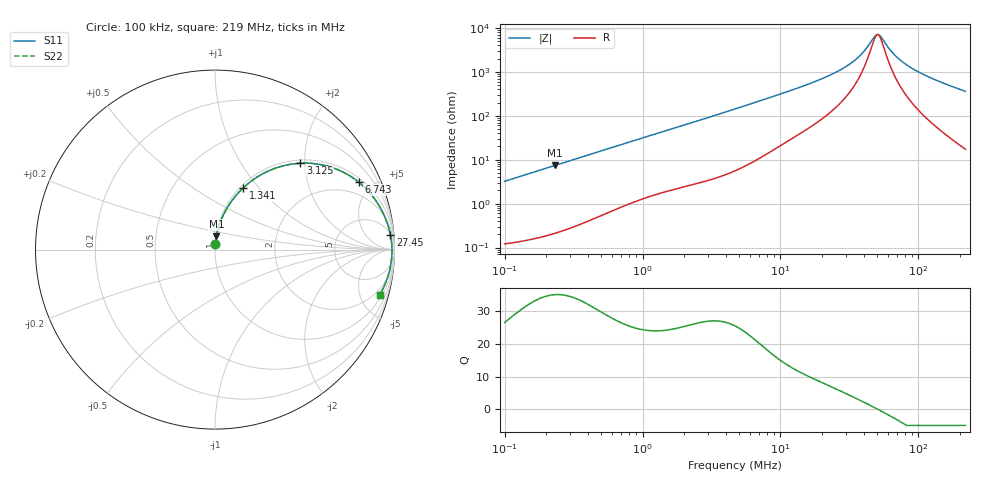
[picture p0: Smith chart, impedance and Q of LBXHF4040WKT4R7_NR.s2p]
! LBXHF4040WKT4R7_NR  S-PARAMETER MODEL  ( General Type )
! Model Generated by TAIYO YUDEN Corporation (http://www.ty-top.com)
! Version 1.0
! TAIYO YUDEN Control No. 210719NI43SB-FBB
! Copyright(c) 2021 TAIYO YUDEN CO.,LTD. All Rights Reserved.
! Product Description (link to TY-COMPAS)
! https://ds.yuden.co.jp/TYCOMPAS/or/detail?pn=LBXHF4040WKT4R7MNR&u=M
! Products Name : Inductors
! Characteristics :
!  Inductance : 4.7 uH , SRF(min) : 36 MHz , DC Resistance(max) : 0.084 Ohm
!  Rated Current : Saturation :2000 mA , Temp Rise : 1500 mA
!  Case Size : 4.0 x 4.0 / 0.157 x 0.157 [mm/inch] , Thickness : 2 / 0.079 [mm/inch]
!  (Conditions: Temperature = 25 degC , DC Bias Current/Voltage = 0A / 0V)
! External Node Assignments :
!  1  o---GGG---o  2
! GND o---------o GND
! Frequency Range : 0.1MHz  -  218.972167MHz  [ 402 STEP ]
# MHz S RI R 50
! Freq[MHz].  S11 Real  S11 Imag  S21 Real  S21 Imag  S12 Real  S12 Imag  S22 Real  S22 Imag
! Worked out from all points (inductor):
!   401 points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, 100 kHz to 219 MHz, reference 50 ohm
!   read as one part in series: L = 5.11 uH near 103.9 kHz
!   highest Q = 35.2 at 233 kHz (marker M1), where L = 5.09 uH
!   self-resonance near 49.82 MHz
!   S11 on the Smith chart (normalised r, x): 100 kHz: 1.00, +0.06; 1.341 MHz: 1.03, +0.83; 3.125 MHz: 1.07, +1.90; 6.743 MHz: 1.20, +4.14; 27.45 MHz: 5, +22; 219 MHz: 1.35, -7.18
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0.1  0.00224 0.0321  0.9978 -0.0321  0.9978 -0.0321  0.00224 0.0321
0.233047  0.00761 0.0739  0.9924 -0.0739  0.9924 -0.0739  0.00761 0.0739
0.362673  0.0165 0.1133  0.9835 -0.1133  0.9835 -0.1133  0.0165 0.1133
0.753099  0.0607 0.2202  0.9393 -0.2202  0.9393 -0.2202  0.0607 0.2202
1.315317  0.1518 0.3386  0.8482 -0.3386  0.8482 -0.3386  0.1518 0.3386
1.340853  0.1564 0.343  0.8436 -0.343  0.8436 -0.343  0.1564 0.343
2.007944  0.2811 0.4302  0.7189 -0.4302  0.7189 -0.4302  0.2811 0.4302
3.124813  0.475 0.4812  0.525 -0.4812  0.525 -0.4812  0.475 0.4812
4.770297  0.6723 0.4501  0.3277 -0.4501  0.3277 -0.4501  0.6723 0.4501
6.743152  0.7996 0.377  0.2004 -0.377  0.2004 -0.377  0.7996 0.377
10.294  0.8967 0.272  0.1033 -0.272  0.1033 -0.272  0.8967 0.272
16.97108  0.9534 0.1648  0.0466 -0.1648  0.0466 -0.1648  0.9534 0.1648
27.44631  0.9772 0.0841  0.0228 -0.0841  0.0228 -0.0841  0.9772 0.0841
37.33357  0.9838 0.0403  0.0162 -0.0403  0.0162 -0.0403  0.9838 0.0403
47.93603  0.9859 0.00702  0.0141 -0.00702  0.0141 -0.00702  0.9859 0.00702
49.81545  0.986 0.00196  0.014 -0.00196  0.014 -0.00196  0.986 0.00196
53.79822  0.9861 -0.00816  0.0139 0.00816  0.0139 0.00816  0.9861 -0.00816
61.54953  0.9856 -0.026  0.0144 0.026  0.0144 0.026  0.9856 -0.026
74.59925  0.9837 -0.0524  0.0163 0.0524  0.0163 0.0524  0.9837 -0.0524
95.78491  0.9784 -0.0894  0.0216 0.0894  0.0216 0.0894  0.9784 -0.0894
138.0275  0.9627 -0.1522  0.0373 0.1522  0.0373 0.1522  0.9627 -0.1522
218.9722  0.9177 -0.2518  0.0823 0.2518  0.0823 0.2518  0.9177 -0.2518
